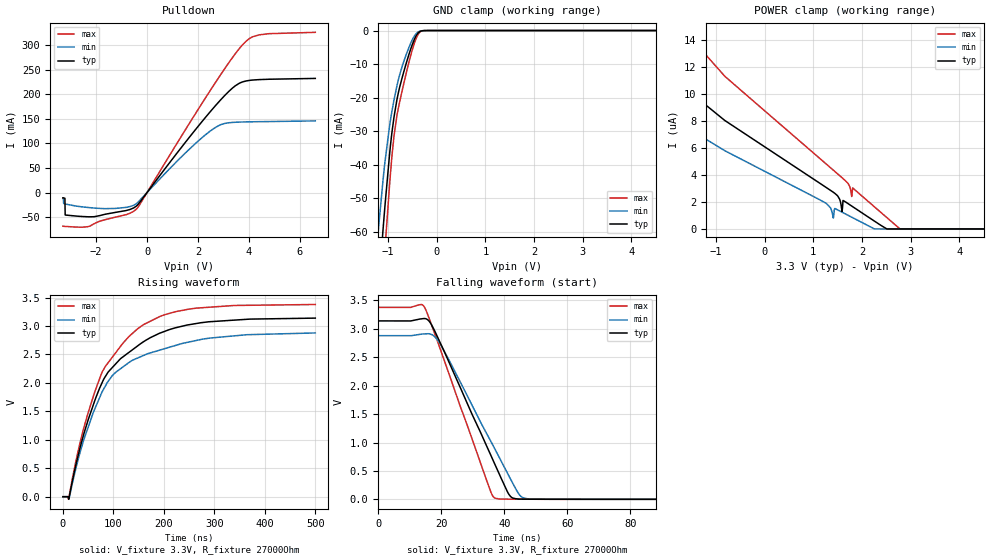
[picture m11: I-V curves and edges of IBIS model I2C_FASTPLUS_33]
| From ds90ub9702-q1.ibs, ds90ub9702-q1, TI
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|   I2C_FastPlus33 Model
[Model]   I2C_FASTPLUS_33
Model_type   I/O_open_drain
Polarity   Non-Inverting
Enable   Active-High
Vinl = 0.99
Vinh = 2.31
Vmeas = 1.65
Vref = 3.3
Cref = 0pF
Rref = 27000
|   typ   min   max
C_comp   1.392003pF   1.392003pF   1.392003pF
[Voltage Range]   3.3   3   3.6
[Temperature Range]   27   105   -40
[Pullup Reference]   3.3   3   3.6
[Pulldown Reference]   -0   0   -0
[Power Clamp Reference]   3.3   3   3.6
[GND Clamp Reference]   0   0   0
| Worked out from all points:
|   slope of the pulldown table from 0 to 0.495 V, typ, clamps not added: 14.5 ohm
|   GND clamp passes 1 mA (typ) near -0.39 V on its own axis
|   falling waveform, V_fixture 3.3V, R_fixture 27000Ohm: 20-80 % time 15.2ns typ, 16.1ns min, 12.9ns max; typ from 3.14 V to 0.002 V
|   rising waveform, V_fixture 3.3V, R_fixture 27000Ohm: 20-80 % time 99.5ns typ, 94.4ns min, 92.4ns max; typ from 0.002 V to 3.14 V
[Pulldown]
|   Voltage   I(typ)   I(min)   I(max)
-3.3V     -10.66mA   -11.81mA   -68.45mA
-3.27V    -10.84mA   -22.15mA   -68.58mA
-3.221V   -11.73mA   -23.04mA   -68.79mA
-3.211V   -45.65mA   -23.2mA    -68.83mA
-2.32V    -49.24mA   -30.33mA   -69.34mA
-1.241V   -40.33mA   -32.32mA   -49.99mA
-419.1mV  -27.53mA   -22.53mA   -33.72mA
2.511V    166.3mA    126.3mA    210.1mA
3.343V    212.1mA    142.6mA    273.8mA
3.907V    227.1mA    143.7mA    308.7mA
4.402V    229.7mA    144.1mA    320.7mA
6.6V      232.1mA    145.7mA    325.8mA
[GND Clamp]
|   Voltage   I(typ)   I(min)   I(max)
-3.3V     -528.6mA   -466.9mA   -595.9mA
-1.211V   -80.34mA   -61.77mA   -97.81mA
-1.102V   -59.67mA   -44.82mA   -73.84mA
-1.063V   -52.53mA   -39.35mA   -65.39mA
-943.8mV  -33.69mA   -26.31mA   -41.91mA
-874.5mV  -25.73mA   -20.64mA   -31.31mA
-815.1mV  -20.61mA   -16.48mA   -25.31mA
-706.2mV  -13.96mA   -10.63mA   -17.82mA
-567.6mV  -7.079mA   -5.004mA   -9.374mA
-458.7mV  -2.703mA   -1.686mA   -3.845mA
-359.7mV  -460.5uA   -270uA     -723.2uA
6.6V      0A         0A         0A
[POWER Clamp]
|   Voltage   I(typ)   I(min)   I(max)
-3.3V     42.87uA    22.78uA    77.21uA
-2.993V   23.33uA    15.21uA    37.79uA
-2.488V   14.76uA    10.86uA    22.03uA
-1.419V   9.829uA    7.138uA    13.8uA
1.254V    3.108uA    1.927uA    4.861uA
1.412V    2.723uA    806.8nA    4.365uA
1.591V    1.287uA    1.246uA    3.805uA
1.61V     2.116uA    1.209uA    3.742uA
1.789V    1.703uA    874.7nA    2.413uA
1.808V    1.656uA    837.6nA    3.045uA
2.779V    0A         0A         7.004nA
6.6V      0A         0A         0A
[Ramp]
R_load = 27000
|   typ   min   max
dV/dt_r   1.88198/9.83865e-08   1.72557/9.39232e-08   2.0256/9.24742e-08
dV/dt_f   1.88329/1.52435e-08   1.72733/1.60789e-08   2.02658/1.29138e-08
[Falling Waveform]
V_fixture = 3.3V
V_fixture_min = 3V
V_fixture_max = 3.6V
R_fixture = 27000Ohm
C_fixture = 0F
|   Time   V(typ)   V(min)   V(max)
0s        3.141V     2.881V     3.379V
14.73ns   3.182V     2.912V     3.378V
16.76ns   3.088V     2.904V     3.095V
19.64ns   2.759V     2.736V     2.652V
35.77ns   771.4mV    1.018V     126.6mV
38.26ns   463.8mV    753.4mV    8.02mV
42.34ns   34.84mV    320mV      4.723mV
45.11ns   5.984mV    61.97mV    4.101mV
48.4ns    3.305mV    8.003mV    3.358mV
500ns     1.787mV    2.013mV    1.579mV
[Rising Waveform]
V_fixture = 3.3V
V_fixture_min = 3V
V_fixture_max = 3.6V
R_fixture = 27000Ohm
C_fixture = 0F
|   Time   V(typ)   V(min)   V(max)
0s        1.787mV    2.013mV    1.579mV
11.21ns   -33.53mV   -5.493mV   -44.53mV
25.56ns   552.8mV    492.9mV    618.9mV
40.04ns   1.058V     962.2mV    1.165V
76.71ns   1.986V     1.824V     2.169V
100.4ns   2.295V     2.152V     2.481V
147.2ns   2.645V     2.435V     2.945V
202.9ns   2.91V      2.605V     3.202V
273.1ns   3.057V     2.763V     3.319V
500ns     3.138V     2.878V     3.378V
